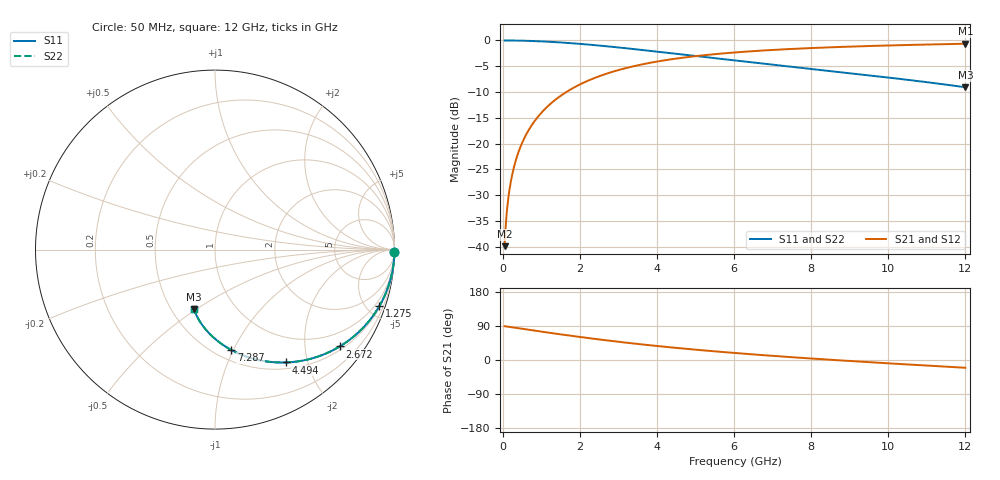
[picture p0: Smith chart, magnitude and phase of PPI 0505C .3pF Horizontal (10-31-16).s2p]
# MHz S MA R 50
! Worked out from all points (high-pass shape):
!   1601 points, 50 MHz to 12 GHz, reference 50 ohm
!   highest |S21| = -0.63 dB at 12 GHz (marker M1); lowest = -39.9 dB at 50 MHz (marker M2)
!   |S21| within 3 dB of the highest: 4.388 GHz to end of sweep
!   lowest |S11| = -9.1 dB at 12 GHz (marker M3), VSWR 2.08, Z = 32.2 - j24.4 ohm
!   |S11| at or under -10 dB: nowhere
!   |S22| runs from -9.1 to 0.0 dB; largest |S21 - S12| = 0
!   S11 on the Smith chart (normalised r, x): 50 MHz: open; 1.275 GHz: 0.59, -5.91; 2.672 GHz: 0.59, -2.81; 4.494 GHz: 0.59, -1.65; 7.287 GHz: 0.60, -0.98; 12 GHz: 0.64, -0.49
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50  0.9999 -0.8  0.01012 89.2  0.01012 89.2  0.9999 -0.8
79.875  0.9999 -1.2  0.01617 88.8  0.01617 88.8  0.9999 -1.2
139.625  0.9996 -2.1  0.02826 87.9  0.02826 87.9  0.9996 -2.1
199.375  0.9992 -3.0  0.04033 87.0  0.04033 87.0  0.9992 -3.0
244.1875  0.9988 -3.7  0.04937 86.3  0.04937 86.3  0.9988 -3.7
296.4688  0.9982 -4.5  0.05991 85.5  0.05991 85.5  0.9982 -4.5
415.9688  0.9964 -6.3  0.0839 83.7  0.0839 83.7  0.9964 -6.3
572.8125  0.9933 -8.7  0.1152 81.3  0.1152 81.3  0.9933 -8.7
767  0.9881 -11.6  0.1534 78.4  0.1534 78.4  0.9881 -11.6
998.5312  0.9801 -15.0  0.198 75.0  0.198 75.0  0.9801 -15.0
1274.875  0.9681 -19.0  0.2495 70.9  0.2495 70.9  0.9681 -19.0
1633.375  0.9493 -24.1  0.3132 65.8  0.3132 65.8  0.9493 -24.1
2044.156  0.924 -29.7  0.3811 60.2  0.3811 60.2  0.924 -29.7
2671.531  0.88 -37.8  0.4732 52.1  0.4732 52.1  0.88 -37.8
3328.781  0.8305 -45.6  0.5549 44.3  0.5549 44.3  0.8305 -45.6
4038.312  0.7766 -53.3  0.6275 36.6  0.6275 36.6  0.7766 -53.3
4493.906  0.743 -57.8  0.6667 32.0  0.6667 32.0  0.743 -57.8
6025  0.6395 -71.3  0.7653 18.4  0.7653 18.4  0.6395 -71.3
7287.219  0.5666 -80.8  0.8199 8.9  0.8199 8.9  0.5666 -80.8
8019.156  0.5286 -85.8  0.8444 3.8  0.8444 3.8  0.5286 -85.8
10013.31  0.4364 -98.2  0.8943 -8.9  0.8943 -8.9  0.4364 -98.2
12000  0.3515 -109.6  0.9295 -20.5  0.9295 -20.5  0.3515 -109.6
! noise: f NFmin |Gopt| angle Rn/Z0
50  0.002885  0.9899  0.7411  0.06566
1372  0.006153  0.8112  10.42  0.006741
2701  0.009111  0.7357  15.16  0.006772
4031  0.01181  0.694  19.45  0.007317
5360  0.01436  0.6674  23.65  0.007955
6682  0.01684  0.6497  27.78  0.008629
8012  0.01932  0.638  31.87  0.009342
9341  0.02182  0.6309  35.86  0.0101
1.067e+04  0.02439  0.6274  39.76  0.01092
1.2e+04  0.02705  0.627  43.54  0.01182
